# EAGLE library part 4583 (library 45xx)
Dual SCHMITT TRIGGER
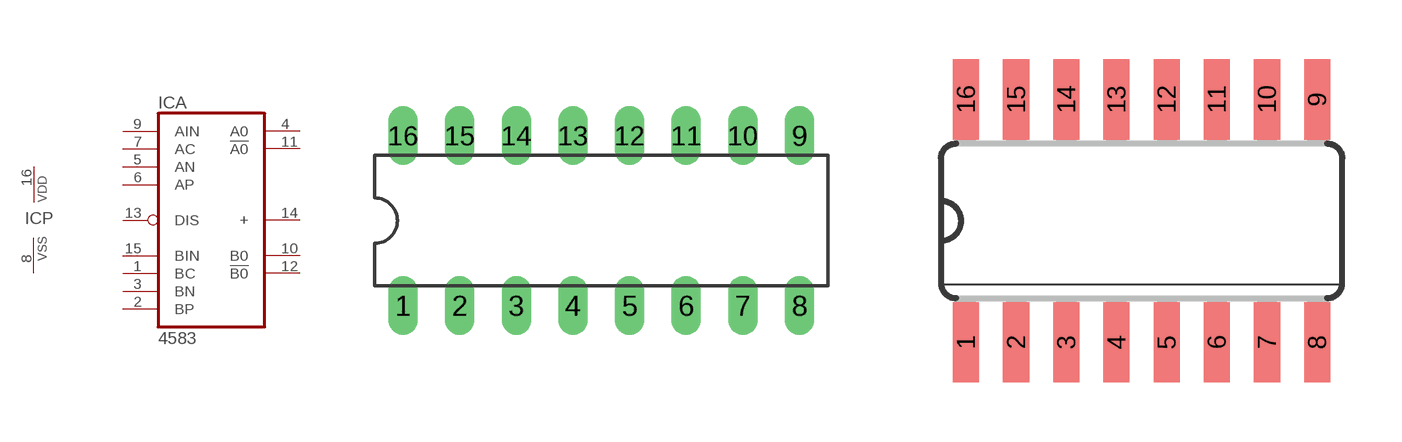
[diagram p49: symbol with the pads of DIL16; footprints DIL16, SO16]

Designator prefix IC; gates A=4583 P=PWRN

## 4583N  [DIL16]
1  A:BC  in
2  A:BP  in
3  A:BN  in
4  A:A0  out
5  A:AN  in
6  A:AP  in
7  A:AC  in
8  P:VSS  pwr
9  A:AIN  in
10  A:B0  out
11  A:!A0  out
12  A:!B0  out
13  A:DIS  in
14  A:+  out
15  A:BIN  in
16  P:VDD  pwr

## 4583D  [SO16]
Pads as for DIL16

## Footprint DIL16 (pad centres in mm)
Dual In Line Package
drill 0.813 long: 1 -8.89,-3.81; 2 -6.35,-3.81; 3 -3.81,-3.81; 4 -1.27,-3.81; 5 1.27,-3.81; 6 3.81,-3.81; 7 6.35,-3.81; 8 8.89,-3.81; 9 8.89,3.81; 10 6.35,3.81; 11 3.81,3.81; 12 1.27,3.81; 13 -1.27,3.81; 14 -3.81,3.81; 15 -6.35,3.81; 16 -8.89,3.81

## Footprint SO16 (pad centres in mm)
Small Outline package 150 mil
smd 0.66 x 2.032: 1 -4.445,-3.073; 2 -3.175,-3.073; 3 -1.905,-3.073; 4 -0.635,-3.073; 5 0.635,-3.073; 6 1.905,-3.073; 7 3.175,-3.073; 8 4.445,-3.073; 9 4.445,3.073; 10 3.175,3.073; 11 1.905,3.073; 12 0.635,3.073; 13 -0.635,3.073; 14 -1.905,3.073; 15 -3.175,3.073; 16 -4.445,3.073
